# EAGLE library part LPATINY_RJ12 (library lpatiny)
CORCOM Modular RJ Jacks No Shield Source: www.tycoelectronics.com .. ENG_DS_1654001_1099_RJ_L_0507.pdf
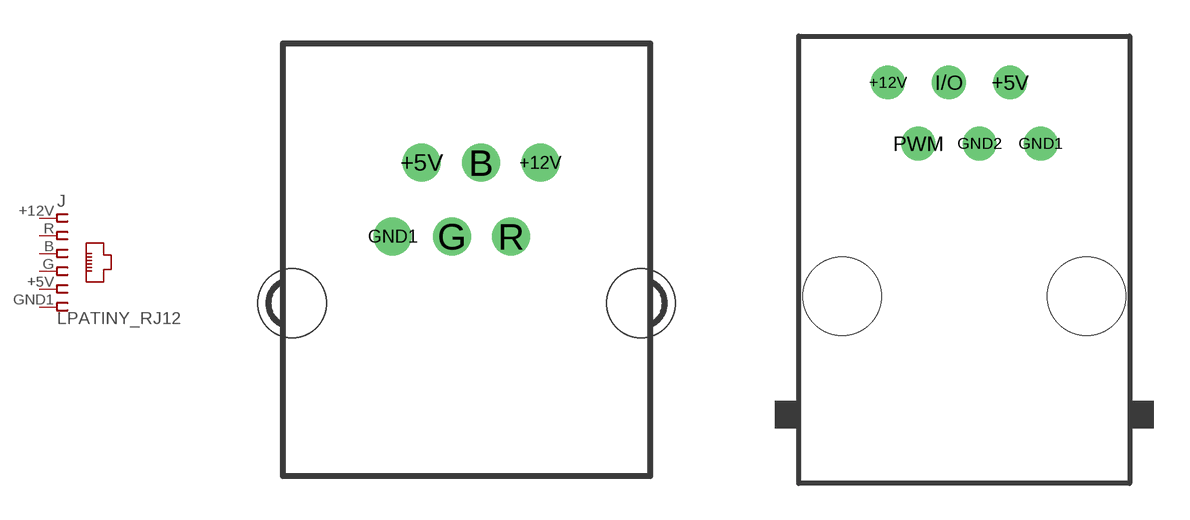
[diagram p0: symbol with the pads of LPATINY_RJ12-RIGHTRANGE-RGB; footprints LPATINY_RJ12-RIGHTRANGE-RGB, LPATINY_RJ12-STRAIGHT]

Designator prefix J

## LPATINY_RJ12RIGHTANGLE-RGB  [LPATINY_RJ12-RIGHTRANGE-RGB]
+5V  5  pwr
+12V  1  pwr
B  3
G  4  pwr
GND1  6  pwr
R  2

## LPATINY_RJ12STRAIGHT  [LPATINY_RJ12-STRAIGHT]
+5V  5  pwr
+12V  1  pwr
GND1  6  pwr
GND2  4  pwr
I/O  3
PWM  2

## LPATINY_RJ12STRAIGHT-ANALOG  [LPATINY_RJ12-STRAIGHT-ANALOG]
+5V  5  pwr
+12V  1  pwr
GND1  6  pwr
GND2  4  pwr
GND3  2
IN  3

## LPATINY_RJ12STRAIGHT-I2C  [LPATINY_RJ12-STRAIGHT-I2C]
+5V  5  pwr
+12V  1  pwr
GND1  6  pwr
GND2  4  pwr
SCL  2
SDA  3

## LPATINY_RJ12STRAIGHT-RGB  [LPATINY_RJ12-STRAIGHT-RGB]
Pads as for LPATINY_RJ12-RIGHTRANGE-RGB

## LPATINY_RJ12STRAIGHT-RS232-SERVER  [LPATINY_RJ12-STRAIGHT-RS232]
+5V  5  pwr
+12V  1  pwr
GND1  6  pwr
GND2  4  pwr
RX  2
TX  3

## Footprint LPATINY_RJ12-RIGHTRANGE-RGB (pad centres in mm)
drill 0.8 pad 1.3: +5V -1.54,4.84; +12V 2.54,4.84; B 0.5,4.84; G -0.5,2.3; GND1 -2.54,2.3; R 1.54,2.3
hole 2.36 at -6,0
hole 2.36 at 6,0

## Footprint LPATINY_RJ12-STRAIGHT (pad centres in mm)
RJ11 Low Profile No Shield For all RJ11 N and Z Series Models Source: www.tycoelectronics.com .. ENG_DS_1654001_1099_RJ_L_0507.pdf
drill 0.9 pad 1.4: +5V 1.905,8.89; +12V -3.175,8.89; GND1 3.175,6.35; GND2 0.635,6.35; I/O -0.635,8.89; PWM -1.905,6.35
hole 3.251 at -5.08,0
hole 3.251 at 5.08,0

## Footprint LPATINY_RJ12-STRAIGHT-ANALOG (pad centres in mm)
drill 0.9 pad 1.4: +5V 1.905,8.89; +12V -3.175,8.89; GND1 3.175,6.35; GND2 0.635,6.35; GND3 -1.905,6.35; IN -0.635,8.89
hole 3.251 at -5.08,0
hole 3.251 at 5.08,0

## Footprint LPATINY_RJ12-STRAIGHT-I2C (pad centres in mm)
drill 0.9 pad 1.4: +5V 1.905,8.89; +12V -3.175,8.89; GND1 3.175,6.35; GND2 0.635,6.35; SCL -1.905,6.35; SDA -0.635,8.89
hole 3.251 at -5.08,0
hole 3.251 at 5.08,0

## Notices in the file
©2009 ROFA.cz - modified and updated by Robert Darlington ‹rdarlington@gmail.com›
